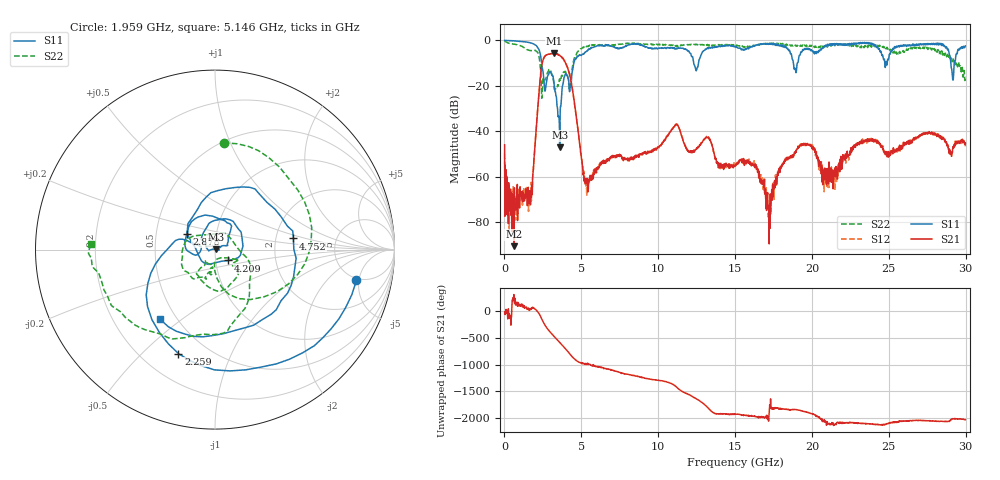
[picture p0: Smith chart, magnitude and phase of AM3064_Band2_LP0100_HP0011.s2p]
# Hz S DB R 50.0
!freq dBS11 angS11 dBS21 angS21 dBS12 angS12 dBS22 angS22
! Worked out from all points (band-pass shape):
!   1600 points, 10 MHz to 29.98 GHz, reference 50 ohm
!   highest |S21| = -5.70 dB at 3.234 GHz (marker M1); lowest = -90.6 dB at 609.8 MHz (marker M2)
!   |S21| within 3 dB of the highest: 2.509 GHz to 3.876 GHz (1.367 GHz wide, 42.8 % of centre)
!   lowest |S11| = -47.1 dB at 3.59 GHz (marker M3), VSWR 1.01, Z = 50.4 + j0.0772 ohm
!   |S11| at or under -10 dB: 2.42 GHz to 4.507 GHz (2.087 GHz wide, 60.2 % of centre); 12.31 GHz to 12.62 GHz (308.9 MHz wide, 2.48 % of centre); 18.8 GHz to 19.05 GHz (254 MHz wide, 1.34 % of centre)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
!   |S22| runs from -25.5 to -0.2 dB; largest |S21 - S12| = 0.017
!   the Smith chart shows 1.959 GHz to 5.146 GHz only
!   S11 on the Smith chart (normalised r, x): 1.959 GHz: 4.72, -4.62; 2.259 GHz: 0.35, -0.65; 2.878 GHz: 0.72, +0.13; 4.209 GHz: 1.15, -0.14; 4.752 GHz: 2.51, +0.39; 5.146 GHz: 0.41, -0.42
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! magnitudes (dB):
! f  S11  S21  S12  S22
! 10 MHz  0.0  -46.0  -49.8  -0.2
! 609.8 MHz  -0.2  -90.6  -67.7  -1.6
! 1.678 GHz  -1.1  -70.1  -69.6  -4.5
! 1.959 GHz  -1.9  -48.9  -49.0  -4.5
! 2.259 GHz  -4.2  -22.0  -21.9  -7.6
! 2.878 GHz  -14.9  -6.0  -6.0  -13.1
! 3.234 GHz  -19.7  -5.7  -5.9  -20.9
! 3.59 GHz  -47.1  -6.7  -6.6  -16.9
! 4.209 GHz  -20.4  -14.3  -14.3  -21.2
! 4.752 GHz  -7.1  -37.7  -37.8  -5.1
! 5.015 GHz  -6.5  -52.2  -51.8  -3.7
! 5.146 GHz  -6.1  -58.3  -58.4  -3.2
! 10 GHz  -3.5  -47.2  -46.9  -1.8
! 11.2 GHz  -3.6  -37.1  -37.1  -2.4
! 15 GHz  -2.7  -54.9  -54.7  -2.0
! 16.34 GHz  -2.3  -54.6  -55.3  -2.4
! 17.25 GHz  -1.5  -71.9  -74.6  -1.2
! 18.19 GHz  -2.3  -54.1  -53.3  -1.9
! 19.99 GHz  -4.4  -46.8  -46.7  -2.2
! 20.95 GHz  -2.4  -63.5  -58.4  -2.4
! 25 GHz  -7.9  -51.4  -49.7  -3.4
! 29.98 GHz  -2.4  -45.4  -46.6  -15.8
